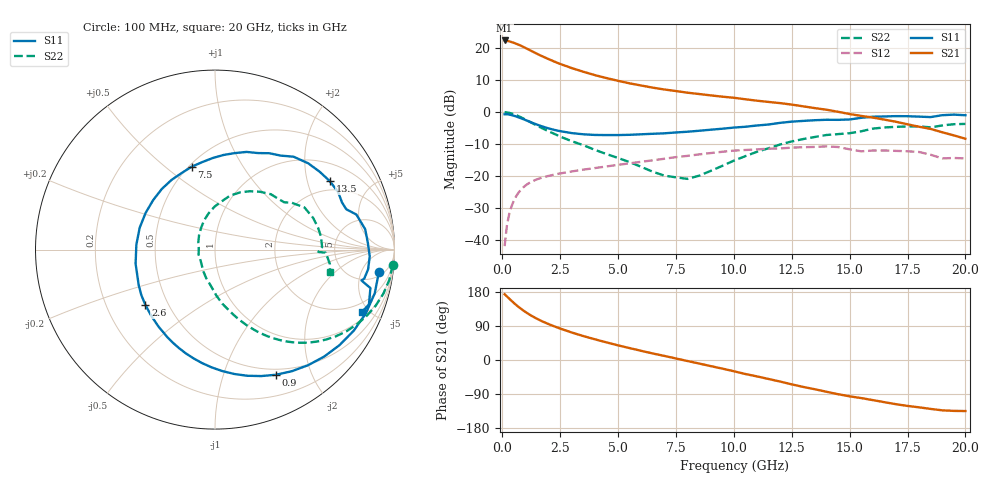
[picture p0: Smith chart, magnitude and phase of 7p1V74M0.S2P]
! Infineon Technologies  Discrete & RF Semiconductors
! bfp620
! VCE =  1.7 V,  IC =  4.0 mA
! Common Emitter S-Parameters:  Sep 2002
# GHz  S  MA  R  50
!  f  S11  S21  S12  S22
! GHz  MAG  ANG  MAG  ANG  MAG  ANG  MAG  ANG
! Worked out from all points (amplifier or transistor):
!   59 points, 100 MHz to 20 GHz, reference 50 ohm
!   highest |S21| = 22.3 dB at 100 MHz (marker M1)
!   |S21| within 3 dB of that: start of sweep to 1.181 GHz
!   unconditionally stable (mu >= 1): 5.087 GHz to 11.89 GHz; 14.59 GHz to 15.46 GHz; 17.2 GHz to end of sweep
!   at 1 GHz: K = 0.27, MSG = 21.5 dB, |S12| = -22.9 dB
!   at 5.5 GHz: K = 1.03, MAG = 11.4 dB, |S12| = -16.0 dB
!   at 20 GHz: K = 1.38, MAG = -0.6 dB, |S12| = -14.5 dB
!   S11 on the Smith chart (normalised r, x): 100 MHz: 6, -11; 900 MHz: 0.43, -1.51; 2.6 GHz: 0.37, -0.31; 7.5 GHz: 0.52, +0.62; 13.5 GHz: 1.62, +2.77; 20 GHz: 1.37, -4.57
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0.1  0.9217 -7.8  13.05 173.4  0.0081 83.2  0.9937 -5.0
0.3  0.9124 -22.9  12.62 161.9  0.0258 77.9  0.97 -14.6
0.5  0.8745 -37.5  11.97 150.5  0.0416 70.0  0.9219 -23.7
0.7  0.8268 -51.2  11.22 140.2  0.0552 62.8  0.8618 -31.9
0.9  0.7758 -64.0  10.39 131.0  0.0665 56.4  0.7964 -39.0
1.1  0.7253 -75.7  9.562 122.8  0.0757 50.9  0.731 -45.2
1.3  0.6782 -86.5  8.779 115.4  0.0832 46.3  0.6692 -50.4
1.6  0.6176 -101.2  7.763 105.7  0.092 40.7  0.5878 -56.9
2  0.5556 -118.5  6.681 94.8  0.1009 35.3  0.5008 -63.7
2.6  0.4957 -141.4  5.447 80.8  0.1118 29.3  0.4009 -72.0
3  0.4692 -154.9  4.839 72.5  0.1184 26.1  0.3508 -76.7
3.5  0.4493 -169.9  4.244 63.2  0.1264 22.7  0.3039 -82.3
5  0.4373 152.0  3.064 38.6  0.1501 13.9  0.192 -99.1
6  0.4494 131.3  2.588 24.2  0.1675 7.9  0.1396 -117.0
7  0.4656 113.3  2.244 10.8  0.1868 1.7  0.102 -141.3
7.5  0.4799 105.7  2.123 4.0  0.1982 -2.1  0.0958 -162.3
10.5  0.5891 65.9  1.58 -37.0  0.2559 -29.3  0.2052 100.0
12  0.6778 49.8  1.376 -56.9  0.2705 -43.2  0.3118 74.5
13.5  0.7448 30.8  1.15 -77.2  0.2858 -58.6  0.4085 52.1
15  0.7651 17.1  0.93 -95.8  0.2621 -78.4  0.4673 34.3
17  0.8629 -2.5  0.705 -116.6  0.2478 -89.3  0.587 12.0
20  0.8905 -22.8  0.383 -134.7  0.1892 -104.8  0.6526 -10.9
